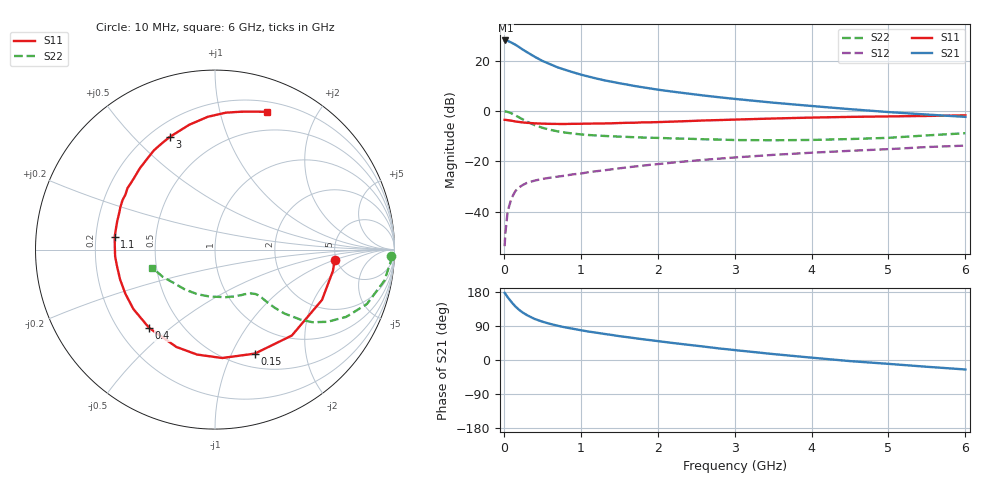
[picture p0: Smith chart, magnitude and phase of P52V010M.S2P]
! SIEMENS Small Signal Semiconductors
! BFP183
! Si NPN RF Bipolar Junction Transistor in SOT143
! VCE = 2 V  IC = 10 mA
! Common Emitter S-Parameters:  March  1996
# GHz  S  MA  R  50
!  f  S11  S21  S12  S22
! GHz  MAG  ANG  MAG  ANG  MAG  ANG  MAG  ANG
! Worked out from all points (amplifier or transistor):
!   36 points, 10 MHz to 6 GHz, reference 50 ohm
!   highest |S21| = 28.0 dB at 20 MHz (marker M1)
!   |S21| within 3 dB of that: start of sweep to 216.3 MHz
!   unconditionally stable (mu >= 1): 1.13 GHz to 5.671 GHz
!   at 250 MHz: K = 0.33, MSG = 26.8 dB, |S12| = -29.2 dB
!   at 1.4 GHz: K = 1.09, MAG = 15.5 dB, |S12| = -23.1 dB
!   at 6 GHz: K = 0.95, MSG = 5.7 dB, |S12| = -13.7 dB
!   lowest NFmin = 1.30 dB at 450 MHz
!   S11 on the Smith chart (normalised r, x): 10 MHz: 4.81, -1.04; 150 MHz: 0.65, -1.23; 400 MHz: 0.33, -0.42; 1.1 GHz: 0.28, +0.06; 3 GHz: 0.28, +0.64; 6 GHz: 0.30, +1.40
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0.01  0.6691 -5.1  24.86 177.2  0.0021 81.6  0.9839 -2.0
0.02  0.6676 -10.3  25 174.6  0.0038 83.0  0.9805 -4.2
0.05  0.6588 -25.2  24.55 165.7  0.0104 81.0  0.9594 -10.4
0.1  0.6422 -48.2  22.59 152.7  0.0188 68.0  0.8991 -19.7
0.15  0.6206 -69.0  20.57 141.3  0.0259 61.1  0.822 -27.1
0.2  0.6053 -86.2  18.4 132.1  0.0308 55.0  0.7448 -32.7
0.25  0.5933 -99.7  16.33 124.6  0.0345 50.6  0.6769 -36.7
0.3  0.5836 -111.6  14.68 118.5  0.0376 47.2  0.6163 -39.3
0.4  0.5702 -130.0  11.9 108.4  0.0418 43.7  0.5265 -42.6
0.5  0.5626 -143.9  9.858 101.2  0.0451 41.2  0.4659 -44.2
0.6  0.5567 -153.9  8.492 95.4  0.0477 41.1  0.425 -45.0
0.7  0.5543 -162.7  7.325 90.4  0.0501 40.8  0.3952 -45.5
0.9  0.5577 -176.0  5.849 82.4  0.0557 41.5  0.3571 -46.3
1.1  0.5633 172.6  4.821 75.1  0.0613 42.1  0.3347 -47.7
1.5  0.5775 156.0  3.555 63.0  0.0731 43.4  0.3109 -51.9
1.8  0.5957 145.0  2.96 54.9  0.0825 43.5  0.2983 -56.4
2.2  0.6171 132.7  2.414 44.8  0.0951 42.1  0.2866 -63.8
3  0.6761 112.0  1.739 26.2  0.1201 38.1  0.2661 -82.6
3.5  0.7104 101.6  1.464 15.7  0.1351 35.0  0.2633 -96.4
4.5  0.7653 85.5  1.088 -2.9  0.1627 27.5  0.2783 -126.9
5.5  0.7984 74.3  0.851 -17.9  0.1933 20.6  0.3288 -152.6
6  0.8207 69.3  0.765 -25.0  0.2064 16.1  0.363 -163.8
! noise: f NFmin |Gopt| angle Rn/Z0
0.45  1.3  0.15  45  0.18
0.9  1.4  0.2  125  0.19
1.8  2.1  0.34  -170  0.14
